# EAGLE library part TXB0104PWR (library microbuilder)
4-Bit Bi-Directional Level Shifter 1.2V-3.6V (VCCA) to 1.65V-5.5V (VCCB) bi-directional level shifter with auto direction sensing. Max data rate - VCCA 1.8V: 20Mbps (50ns), VCCA 3.3V: 100Mbps (10ns) Digikey: 296-21929-1-ND NOTE: For cheaper alternative see NXP's NTB0104 (Digikey: 568-8404-1-ND)
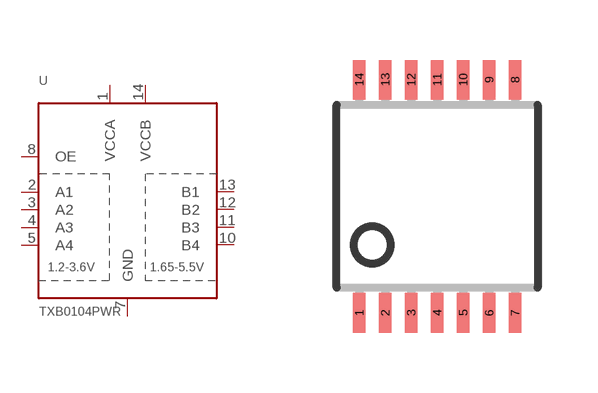
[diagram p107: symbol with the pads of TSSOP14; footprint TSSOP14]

Designator prefix U

## TXB0104PWR  [TSSOP14]
1  VCCA
2  A1
3  A2
4  A3
5  A4
7  GND
8  OE
10  B4
11  B3
12  B2
13  B1
14  VCCB

## Footprint TSSOP14 (pad centres in mm)
Thin Shrink Small Outline Plastic 14
smd 0.305 x 0.991: 1 -1.95,-2.918; 2 -1.3,-2.918; 3 -0.65,-2.918; 4 0,-2.918; 5 0.65,-2.918; 6 1.3,-2.918; 7 1.95,-2.918; 8 1.95,2.918; 9 1.3,2.918; 10 0.65,2.918; 11 0,2.918; 12 -0.65,2.918; 13 -1.3,2.918; 14 -1.95,2.918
